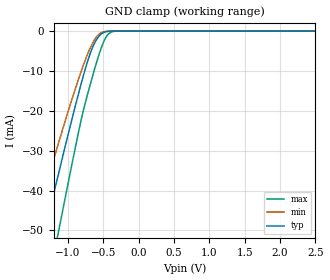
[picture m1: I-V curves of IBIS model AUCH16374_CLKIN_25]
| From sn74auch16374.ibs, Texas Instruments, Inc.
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[Model]   AUCH16374_CLKIN_25
Model_type  Input
Vinl=0.7
Vinh=1.7
| variable   typ   min   max
C_comp   2.38pF   1.92pF   2.72pF
[Temperature Range]   40   100   -40
| Ambient temperature   25   85   -40
[Voltage range]   2.5   2.3   2.7
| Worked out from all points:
|   GND clamp passes 1 mA (typ) near -0.55 V on its own axis
[GND Clamp]
| AUCH16374_CLKIN_25
|   Voltage   I(typ)   I(min)   I(max)
-3.6V     -222.3mA   -186.1mA   -267.5mA
-1.49V    -62.29mA   -49.79mA   -82.1mA
-1.35V    -51.8mA    -41.14mA   -69.63mA
-1.305V   -48.45mA   -38.39mA   -65.61mA
-1.17V    -38.46mA   -30.25mA   -53.55mA
-1.12V    -34.79mA   -27.28mA   -49.08mA
-735mV    -8.324mA   -6.331mA   -16.67mA
-635mV    -3.426mA   -2.471mA   -10.25mA
-525mV    -682.5uA   -360.4uA   -4.021mA
-430mV    -73.19uA   -34.73uA   -776.9uA
-325mV    -3.339uA   -2.006uA   -30.74uA
2.5V      313.9pA    400.9pA    470.4pA
